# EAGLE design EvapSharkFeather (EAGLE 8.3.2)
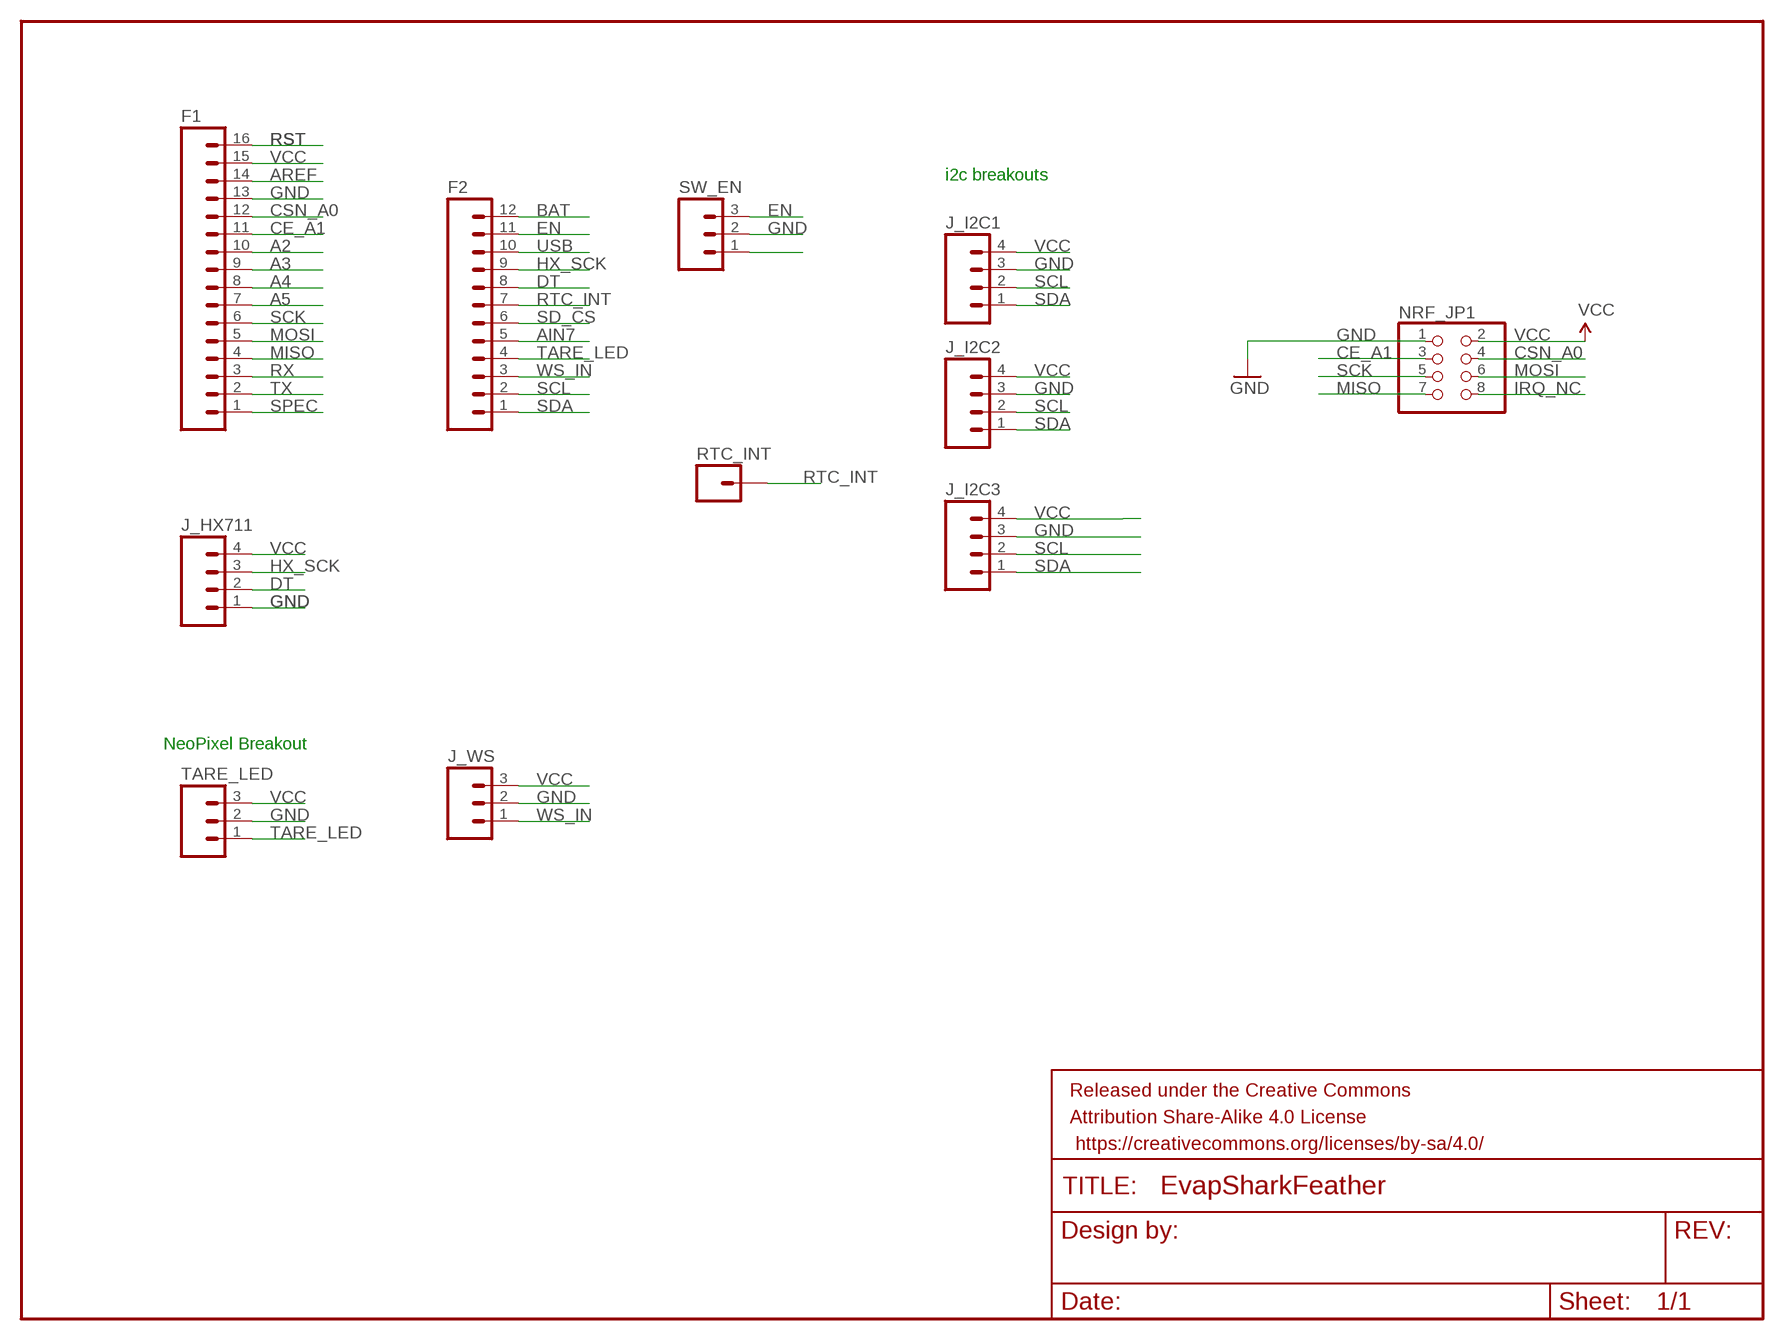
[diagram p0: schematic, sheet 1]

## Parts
F1  M16PTH  [1X16]
F2  M12PTH  [1X12]
FRAME1  FRAME-LETTER  [CREATIVE_COMMONS]
J_HX711  M04PTH  [1X04]
J_I2C1  M04PTH  [1X04]
J_I2C2  M04PTH  [1X04]
J_I2C3  M04PTH  [1X04]
J_WS  M03PTH  [1X03]
NRF_JP1  PINHD-2X4  [2X04]
RTC_INT  M01PTH  [1X01]
SW_EN  M03PTH  [1X03]
TARE_LED  M03PTH  [1X03]

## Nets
A2: F1.10
A3: F1.9
A4: F1.8
A5: F1.7
AIN7: F2.5
AREF: F1.14
BAT: F2.12
CE_A1: F1.11 NRF_JP1.3
CSN_A0: F1.12 NRF_JP1.4
DT: F2.8 J_HX711.2
EN: F2.11 SW_EN.3
GND: F1.13 J_HX711.1 J_I2C1.3 J_I2C2.3 J_I2C3.3 J_WS.2 NRF_JP1.1 SW_EN.2 TARE_LED.2
HX_SCK: F2.9 J_HX711.3
IRQ_NC: NRF_JP1.8
MISO: F1.4 NRF_JP1.7
MOSI: F1.5 NRF_JP1.6
N$3: SW_EN.1
RST: F1.16
RTC_INT: F2.7 RTC_INT.1
RX: F1.3
SCK: F1.6 NRF_JP1.5
SCL: F2.2 J_I2C1.2 J_I2C2.2 J_I2C3.2
SD_CS: F2.6
SDA: F2.1 J_I2C1.1 J_I2C2.1 J_I2C3.1
SPEC: F1.1
TARE_LED: F2.4 TARE_LED.1
TX: F1.2
USB: F2.10
VCC: F1.15 J_HX711.4 J_I2C1.4 J_I2C2.4 J_I2C3.4 J_WS.3 NRF_JP1.2 TARE_LED.3
WS_IN: F2.3 J_WS.1

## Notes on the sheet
- i2c breakouts
- NeoPixel Breakout

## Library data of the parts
F1 = SparkFun-Connectors:M16: 1x16 .1" header
F2 = SparkFun-Connectors:M12: Header 12 Standard 12-pin 0.1" header. Use with straight break away headers (SKU : PRT-00116), right angle break away headers (PRT-00553), swiss pins (PRT-00743), machine pins (PRT-00117), and female headers (PRT-00115).
FRAME1 = SparkFun-Aesthetics:FRAME-LETTER: Schematic Frame
J_HX711 J_I2C1-J_I2C3 = SparkFun-Connectors:M04: Header 4 Standard 4-pin 0.1" header. Use with straight break away headers (SKU : PRT-00116), right angle break away headers (PRT-00553), swiss pins (PRT-00743), machine pins (PRT-00117), and female headers (PRT-00115). Molex polarized connector foot print use with SKU : PRT-08231 with associated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; PROD_ID: CONN-09696
J_WS SW_EN TARE_LED = SparkFun-Connectors:M03: Header 3 Standard 3-pin 0.1" header. Use with straight break away headers (SKU : PRT-00116), right angle break away headers (PRT-00553), swiss pins (PRT-00743), machine pins (PRT-00117), and female headers (PRT-00115). Molex polarized connector foot print use with SKU : PRT-08232 with associated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
NRF_JP1 = pinhead:PINHD-2X4: PIN HEADER
RTC_INT = SparkFun-Connectors:M01: Header 1

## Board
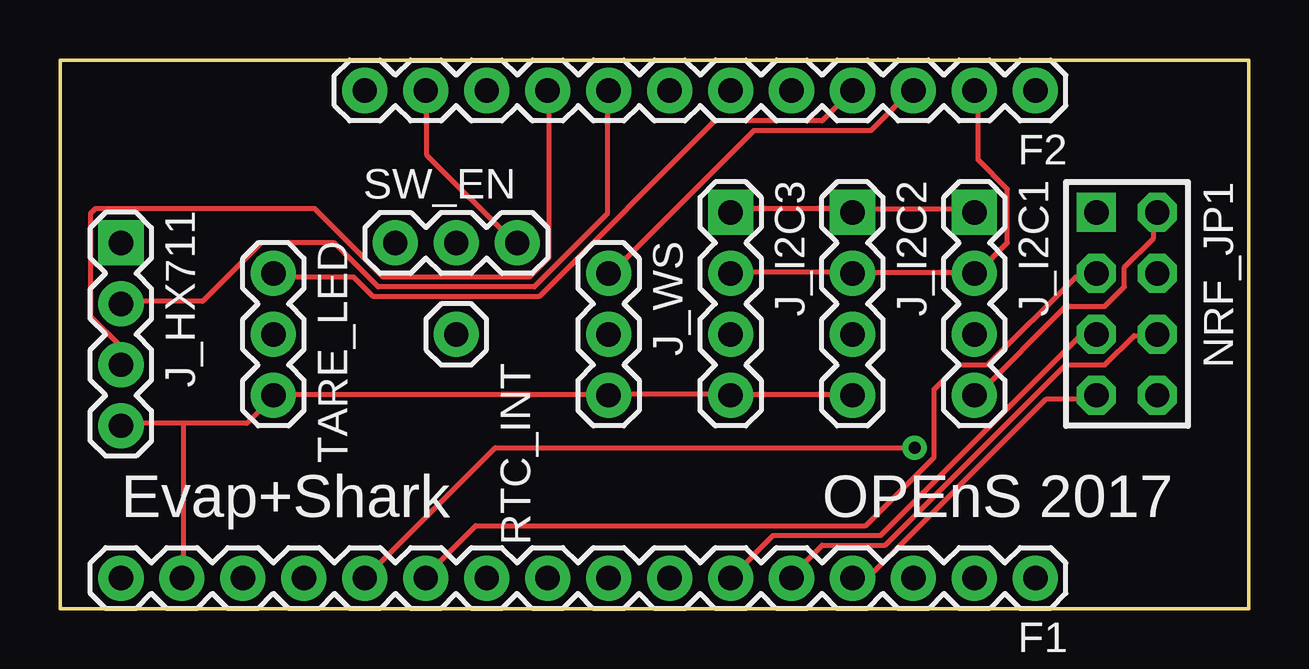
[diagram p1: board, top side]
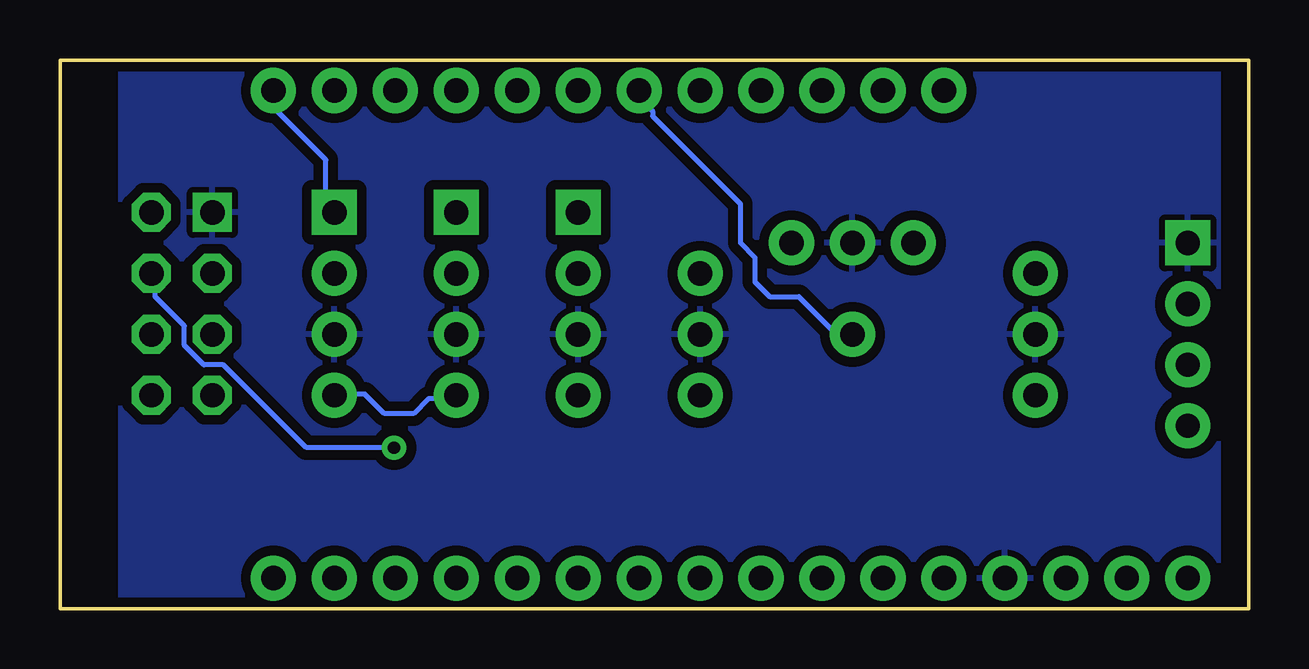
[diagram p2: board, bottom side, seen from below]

Size 49.53 x 22.86 mm. Coordinates in mm from the lower left corner, seen from the top.
Outline: 0,0 0,22.86 49.53,22.86 49.53,0 0,0
Copper layers (1*16): Top 0.035mm / dielectric 1.5mm / Bottom 0.035mm
Design rules "SparkFun": minimum track width 8mil, minimum drill 20mil, track to track 8mil, track to pad 8mil, pad to pad 8mil, via to via 8mil, smd to smd 8mil, copper to edge 8mil, drill to drill 8mil, minimum pad ring 12mil, minimum via ring 10mil, stop-mask expansion 4mil, vias tented up to drill 20mil, thermal gap 10mil

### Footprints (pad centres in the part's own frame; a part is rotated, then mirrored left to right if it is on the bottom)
1X16 = drill 1.016 pad 1.88: 1 0,0; 2 2.54,0; 3 5.08,0; 4 7.62,0; 5 10.16,0; 6 12.7,0; 7 15.24,0; 8 17.78,0; 9 20.32,0; 10 22.86,0; 11 25.4,0; 12 27.94,0; 13 30.48,0; 14 33.02,0; 15 35.56,0; 16 38.1,0
1X12 = drill 1.016 pad 1.88: 1 0,0; 2 2.54,0; 3 5.08,0; 4 7.62,0; 5 10.16,0; 6 12.7,0; 7 15.24,0; 8 17.78,0; 9 20.32,0; 10 22.86,0; 11 25.4,0; 12 27.94,0
1X04 = drill 1.016 pad 1.88 square: 1 0,0 | drill 1.016 pad 1.88: 2 2.54,0; 3 5.08,0; 4 7.62,0
1X03 = drill 1.016 pad 1.88: 1 0,0; 2 2.54,0; 3 5.08,0
2X04 = drill 1.016 square: 1 -3.81,-1.27 | drill 1.016 octagon: 2 -3.81,1.27; 3 -1.27,-1.27; 4 -1.27,1.27; 5 1.27,-1.27; 6 1.27,1.27; 7 3.81,-1.27; 8 3.81,1.27
1X01 = drill 1.016 pad 1.88: 1 0,0

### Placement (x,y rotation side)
F1  40.64,1.27 180 top
F2  40.64,21.59 180 top
FRAME1  not placed on the board
J_HX711  2.54,15.24 270 top
J_I2C1  38.1,16.51 270 top
J_I2C2  33.02,16.51 270 top
J_I2C3  27.94,16.51 270 top
J_WS  22.86,13.97 270 top
NRF_JP1  44.45,12.7 270 top
RTC_INT  16.51,11.43 270 top
SW_EN  13.97,15.24 0 top
TARE_LED  8.89,13.97 270 top

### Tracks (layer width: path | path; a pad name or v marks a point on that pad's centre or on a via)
CE_A1
  Top 0.203: NRF_JP1.3 43.13,13.82 42.32,13.82 38.66,10.16 37.44,10.16 36.42,9.14 36.42,6.3 33.58,3.45 17.32,3.45 15.29,1.42 F1.11
CSN_A0  (via drill 0.51)
  Top 0.203: v35.61,6.71 18.14,6.71 F1.12
  Bottom 0.203: v35.61,6.71 39.27,6.71 42.72,10.16 43.54,10.16 44.35,10.97 44.35,11.79 45.57,13.01 45.57,13.82 NRF_JP1.4
DT
  Top 0.203: J_HX711.2 2.69,12.8 5.94,12.8 8.38,15.24 11.43,15.24 13.26,13.41 19.76,13.41 22.81,16.46 22.81,21.54 F2.8
EN
  Top 0.203: F2.11 15.29,21.54 15.29,18.9 18.95,15.24 SW_EN.3
GND
  pour Bottom (isolate 0.406): 1.27,0 1.27,22.86 46.99,22.86 46.99,0
HX_SCK
  Top 0.203: J_HX711.3 2.49,10.16 2.49,10.97 1.27,12.19 1.27,16.46 1.47,16.66 10.62,16.66 13.46,13.82 19.56,13.82 20.37,14.63 20.37,21.54 F2.9
MISO
  Top 0.203: NRF_JP1.7 43.13,8.74 41.1,8.74 33.78,1.42 33.17,1.42 F1.4
MOSI
  Top 0.203: NRF_JP1.6 45.57,11.38 44.75,11.38 43.54,10.16 41.91,10.16 34.39,2.64 31.75,2.64 30.53,1.42 F1.5
RTC_INT
  Bottom 0.203: RTC_INT.1 16.51,11.58 17.32,11.58 18.75,13.01 19.96,13.01 20.57,13.61 20.57,14.63 21.18,15.24 21.18,16.87 24.84,20.52 24.84,20.73 25.25,21.13 25.25,21.54 F2.7
SCK
  Top 0.203: F1.6 29.72,3.05 34.19,3.05 42.52,11.38 43.13,11.38 NRF_JP1.5
SCL
  Top 0.203: J_I2C3.2 28.09,14.02 32.97,14.02 J_I2C2.2 33.17,14.02 38.05,14.02 J_I2C1.2 38.25,14.02 39.47,15.24 39.47,17.48 38.25,18.69 38.25,21.54 F2.2
SDA
  Top 0.203: J_I2C3.1 28.09,16.66 32.97,16.66 J_I2C2.1 33.17,16.66 38.05,16.66 J_I2C1.1
  Bottom 0.203: J_I2C1.1 38.46,16.87 38.46,18.69 40.49,20.73 40.49,21.54 F2.1
TARE_LED
  Top 0.203: F2.4 31.75,20.32 27.28,20.32 19.96,13.01 13.06,13.01 12.24,13.82 8.99,13.82 TARE_LED.1
VCC
  Top 0.203: NRF_JP1.2 45.57,16.46 45.57,15.44 44.35,14.22 44.35,13.41 43.54,12.6 41.91,12.6 38.25,8.94 J_I2C1.4 | J_I2C2.4 32.97,8.94 28.09,8.94 J_I2C3.4 27.89,8.94 23.01,8.94 J_WS.3 22.81,8.94 8.99,8.94 TARE_LED.3 8.79,8.74 7.77,7.72 5.13,7.72 | 5.13,7.72 2.69,7.72 J_HX711.4 | 5.13,7.72 5.13,1.42 F1.15
  Bottom 0.203: J_I2C1.4 38.05,8.94 36.83,8.94 36.02,8.13 34.8,8.13 34.19,8.74 33.17,8.74 J_I2C2.4
WS_IN
  Top 0.203: J_WS.1 23.01,14.02 28.91,19.91 33.78,19.91 35.41,21.54 F2.3

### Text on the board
tPlace: Evap+Shark | OPEnS 2017

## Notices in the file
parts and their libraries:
SparkFun-Aesthetics: Licensing: Creative Commons ShareAlike 4.0 International - https://creativecommons.org/licenses/by-sa/4.0
SparkFun-Aesthetics: Released under the Creative Commons Attribution Share-Alike 4.0 License
SparkFun-Aesthetics: https://creativecommons.org/licenses/by-sa/4.0
